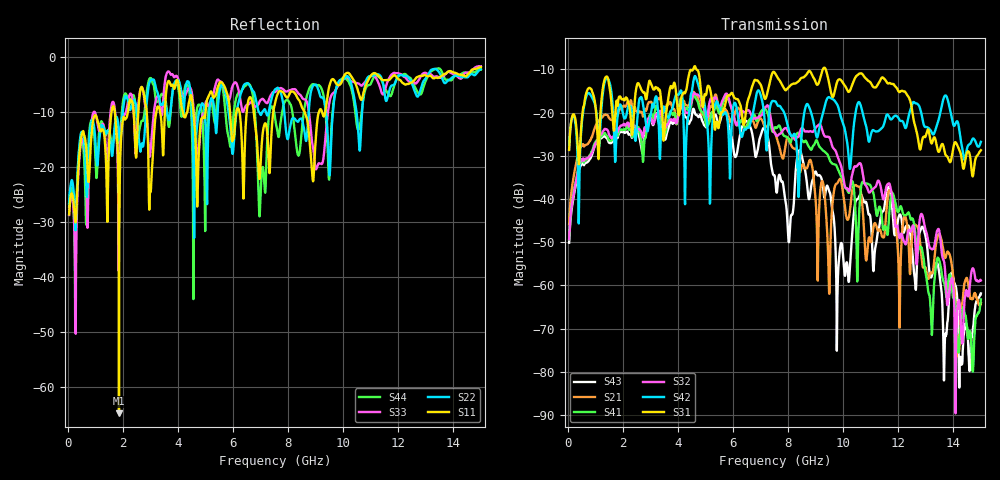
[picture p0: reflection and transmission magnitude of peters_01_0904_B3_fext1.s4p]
# MHZ S RI R 50.00
! FREQ  S11  S12  S13  S14
!  S21  S22  S23  S24
!  S31  S32  S33  S34
!  S41  S42  S43  S44
!  REAL  IMAG  REAL  IMAG  REAL  IMAG  REAL  IMAG
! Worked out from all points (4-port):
!   1496 points, 50 MHz to 15 GHz, reference 50 ohm
!   strongest paths, dB at 50 MHz, 3.79 GHz, 7.53 GHz, 11.27 GHz, 15 GHz:
!     S31: -28.6, -14.4, -10.9, -13.3, -28.7
!     S42: -28.5, -19.2, -17.4, -24.3, -26.7
!     S32: -49.3, -21.7, -24.9, -35.7, -58.8
!     S41: -49.4, -20.3, -23.4, -42.7, -63.2
!     S21: -45.9, -18.7, -24.7, -47.3, -64.1
!     S43: -50.1, -22.4, -35.2, -47.2, -61.8
!   lowest |S11| = -64.8 dB at 1.86 GHz (marker M1), VSWR 1.00, Z = 50 - j0.0563 ohm
!   |S11| at or under -10 dB: start of sweep to 1.592 GHz; 6.751 GHz to 7.464 GHz (712.6 MHz wide, 10 % of centre); 8.596 GHz to 9.125 GHz (529.5 MHz wide, 5.98 % of centre)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
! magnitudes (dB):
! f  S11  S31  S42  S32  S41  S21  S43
! 50 MHz  -28.7  -28.6  -28.5  -49.3  -49.4  -45.9  -50.1
! 1.86 GHz  -64.8  -16.4  -18.6  -23.6  -24.4  -19.6  -24.9
! 7.15 GHz  -12.2  -16.7  -21.9  -19.0  -19.0  -23.3  -23.8
! 9.8 GHz  -5.1  -12.6  -18.3  -30.2  -33.0  -36.2  -59.8
! 11.64 GHz  -4.3  -13.3  -20.6  -36.4  -46.5  -38.7  -37.2
! 14.26 GHz  -3.3  -29.3  -26.1  -67.7  -69.6  -67.9  -76.5
! 15 GHz  -1.9  -28.7  -26.7  -58.8  -63.2  -64.1  -61.8
